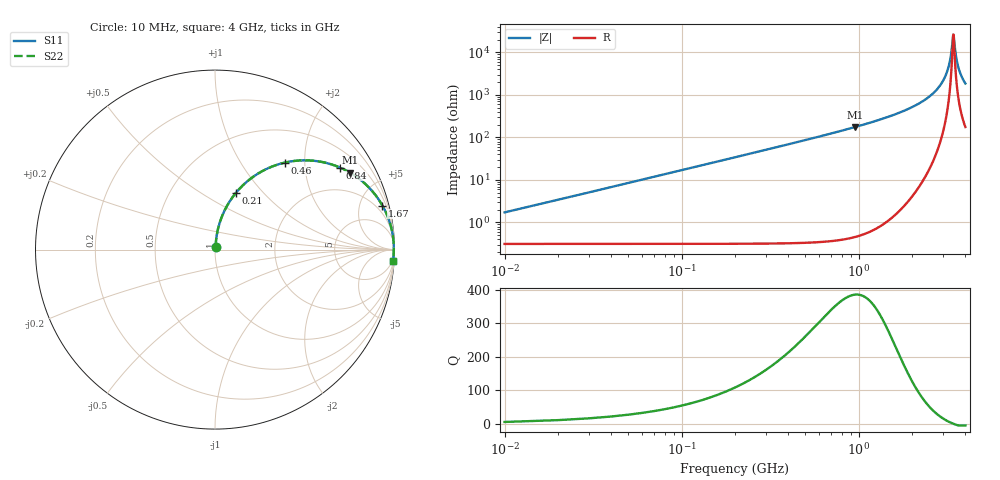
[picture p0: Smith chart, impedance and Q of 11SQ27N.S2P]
! Coilcraft 1111SQ-27N Air Core Inductor
! 16 February 2012
# MHZ S MA R 50
!Freq  MagS11  AngS11  MagS21  AngS21  MagS12  AngS12  MagS22  AngS22
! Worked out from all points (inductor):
!   400 points, 10 MHz to 4 GHz, reference 50 ohm
!   read as one part in series: L = 27 nH near 30 MHz
!   highest Q = 385 at 950 MHz (marker M1), where L = 29.3 nH
!   self-resonance near 3.42 GHz
!   S11 on the Smith chart (normalised r, x): 10 MHz: 1.01, +0.03; 210 MHz: 1.01, +0.72; 460 MHz: 1.01, +1.59; 840 MHz: 1.02, +3.05; 1.67 GHz: 1.08, +7.59; 4 GHz: 3, -30
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10  0.0172 78.6  0.9967 -1.0  0.9967 -1.0  0.0172 78.6
20  0.03397 82.8  0.9963 -1.9  0.9963 -1.9  0.03397 82.8
30  0.0508 83.6  0.9956 -2.9  0.9956 -2.9  0.0508 83.6
70  0.1177 81.7  0.99 -6.8  0.99 -6.8  0.1177 81.7
130  0.2152 76.7  0.9735 -12.4  0.9735 -12.4  0.2152 76.7
210  0.336 69.8  0.9389 -19.7  0.9389 -19.7  0.336 69.8
460  0.6212 51.3  0.7811 -38.5  0.7811 -38.5  0.6212 51.3
680  0.7676 39.6  0.6387 -50.3  0.6387 -50.3  0.7676 39.6
840  0.834 33.2  0.5496 -56.7  0.5496 -56.7  0.834 33.2
950  0.867 29.6  0.4961 -60.3  0.4961 -60.3  0.867 29.6
1340  0.9362 20.2  0.3484 -69.7  0.3484 -69.7  0.9362 20.2
1670  0.9646 14.7  0.2592 -75.0  0.2592 -75.0  0.9646 14.7
2010  0.9806 10.5  0.1882 -79.0  0.1882 -79.0  0.9806 10.5
2670  0.9939 4.5  0.08583 -83.9  0.08583 -83.9  0.9939 4.5
3110  0.9963 1.3  0.03306 -83.2  0.03306 -83.2  0.9963 1.3
3250  0.9964 0.5  0.01811 -78.7  0.01811 -78.7  0.9964 0.5
3340  0.9964 -0.1  0.00916 -67.0  0.00916 -67.0  0.9964 -0.1
3410  0.9962 -0.5  0.00397 -20.0  0.00397 -20.0  0.9963 -0.5
3430  0.9962 -0.6  0.003846 9.6  0.003846 9.6  0.9962 -0.6
3530  0.9959 -1.2  0.01125 68.0  0.01125 68.0  0.996 -1.2
3630  0.9956 -1.8  0.02051 76.4  0.02051 76.4  0.9956 -1.8
4000  0.9935 -3.8  0.05358 80.8  0.05358 80.8  0.9935 -3.8
